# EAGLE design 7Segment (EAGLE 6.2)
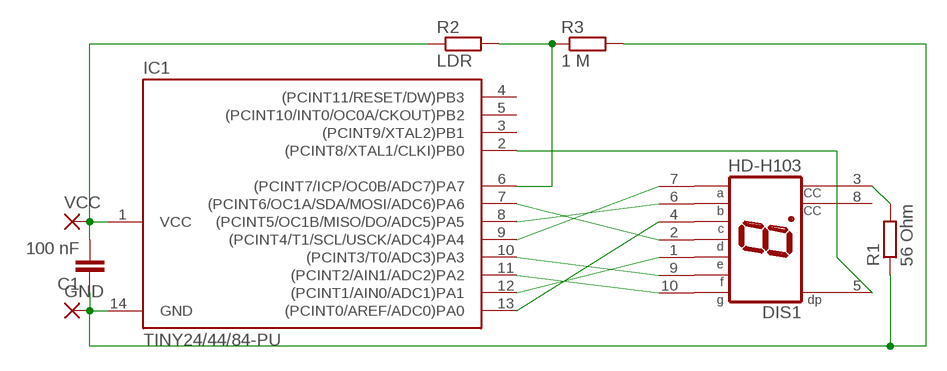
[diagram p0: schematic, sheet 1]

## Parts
C1  100 nF  C-EU025_050-025X075  [C025_050-025X075]
DIS1  HD-H103  [HDSP-M]
GND  2,15/1,0  [2,15/1,0]
IC1  TINY24/44/84-PU  [DIL14]
R1  56 Ohm  R-EU_0207/7  [0207/7]
R2  LDR  R-EU_0204/5  [0204/5]
R3  1 M  R-EU_0207/7  [0207/7]
VCC  2,15/1,0  [2,15/1,0]

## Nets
N$1: DIS1.4(C) IC1.13((PCINT0/AREF/ADC0)PA0)
N$2: C1.1 GND.1(P) IC1.14(GND) R1.1 R3.2
N$3: DIS1.1(E) IC1.12((PCINT1/AIN0/ADC1)PA1)
N$4: DIS1.10(G) IC1.11((PCINT2/AIN1/ADC2)PA2)
N$5: DIS1.9(F) IC1.10((PCINT3/T0/ADC3)PA3)
N$6: DIS1.7(A) IC1.9((PCINT4/T1/SCL/USCK/ADC4)PA4)
N$7: DIS1.6(B) IC1.8((PCINT5/OC1B/MISO/DO/ADC5)PA5)
N$8: DIS1.2(D) IC1.7((PCINT6/OC1A/SDA/MOSI/ADC6)PA6)
N$9: DIS1.5(DP) IC1.2((PCINT8/XTAL1/CLKI)PB0)
N$10: DIS1.3(CC) R1.2
N$12: IC1.6((PCINT7/ICP/OC0B/ADC7)PA7) R2.2 R3.1
VCC: C1.2 IC1.1(VCC) R2.1 VCC.1(P)
Unconnected: DIS1.8(CC) IC1.3((PCINT9/XTAL2)PB1) IC1.4((PCINT11/RESET/DW)PB3) IC1.5((PCINT10/INT0/OC0A/CKOUT)PB2)

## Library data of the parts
C1 = resistor:C-EU: CAPACITOR, European symbol
DIS1 = display-hp:HD-H103: LED DISPLAY 1-character 7 segment, decimal point right
GND VCC = wirepad:2,15/1,0: THROUGH-HOLE PAD
IC1 = avr-5:TINY24/44/84
R1-R3 = resistor:R-EU_: RESISTOR, European symbol

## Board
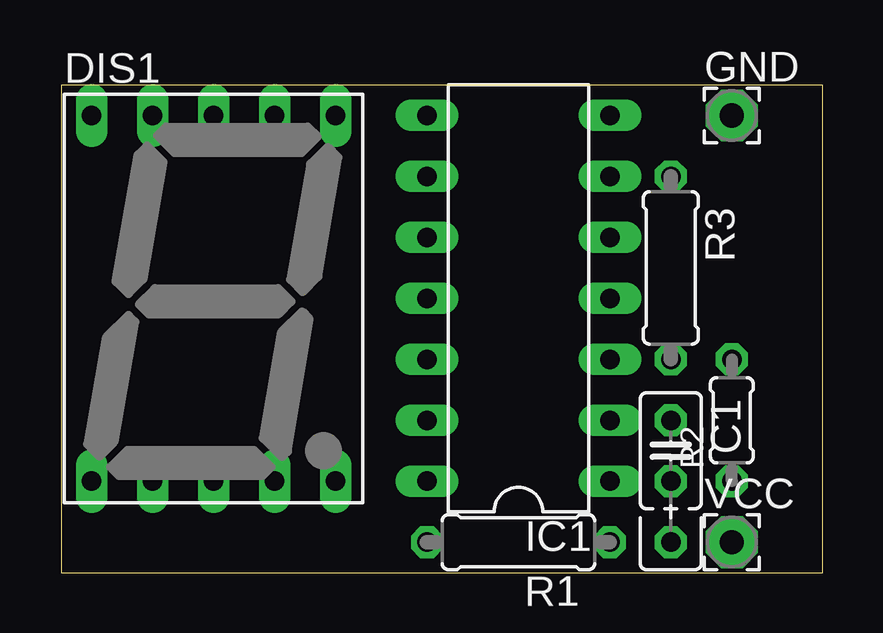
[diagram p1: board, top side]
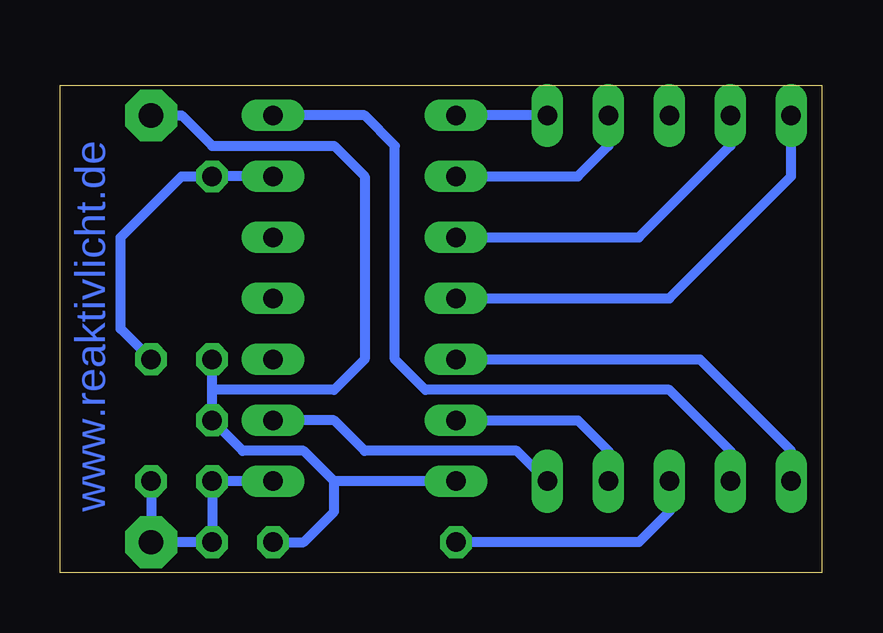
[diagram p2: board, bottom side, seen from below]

Size 31.74 x 20.31 mm. Coordinates in mm from the lower left corner, seen from the top.
Outline: 0,0 31.74,0 31.74,20.31 0,20.31 0,0
Copper layers (1*16): Top 0.035mm / dielectric 1.5mm / Bottom 0.035mm
Design rules: minimum track width 10mil, minimum drill 24mil, track to track 10mil, track to pad 10mil, pad to pad 10mil, via to via 10mil, smd to smd 10mil, copper to edge 40mil, drill to drill 8mil, minimum pad ring 10mil, minimum via ring 8mil, stop-mask expansion 4mil, vias tented up to drill 0mil, thermal gap 10mil

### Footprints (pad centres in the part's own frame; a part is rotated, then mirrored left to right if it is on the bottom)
C025_050-025X075 = drill 0.813 octagon: 1 -1.27,0; 2 1.27,0; 3 3.81,0
HDSP-M = drill 0.813 long: 1 -5.08,-7.62; 2 -2.54,-7.62; 3 0,-7.62; 4 2.54,-7.62; 5 5.08,-7.62; 6 5.08,7.62; 7 2.54,7.62; 8 0,7.62; 9 -2.54,7.62; 10 -5.08,7.62
2,15/1,0 = drill 1.016 pad 2.159 octagon: 1 0,0
DIL14 = drill 0.813 long: 1 -7.62,-3.81; 2 -5.08,-3.81; 3 -2.54,-3.81; 4 0,-3.81; 5 2.54,-3.81; 6 5.08,-3.81; 7 7.62,-3.81; 8 7.62,3.81; 9 5.08,3.81; 10 2.54,3.81; 11 0,3.81; 12 -2.54,3.81; 13 -5.08,3.81; 14 -7.62,3.81
0207/7 = drill 0.813 octagon: 1 -3.81,0; 2 3.81,0
0204/5 = drill 0.813 octagon: 1 -2.54,0; 2 2.54,0

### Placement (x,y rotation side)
C1  25.4,5.08 270 top
DIS1  6.35,11.43 0 top
GND  27.94,19.05 0 top
IC1  19.05,11.43 90 top
R1  19.05,1.27 180 top
R2  27.94,6.35 90 top
R3  25.4,12.7 270 top
VCC  27.94,1.27 0 top

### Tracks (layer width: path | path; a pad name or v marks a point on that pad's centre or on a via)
N$1
  Bottom 0.406: IC1.13 10.16,6.35 8.89,5.08 DIS1.4
N$2
  Bottom 0.406: R1.1 21.59,1.27 20.32,2.54 20.32,3.81 | IC1.14 20.32,3.81 | 20.32,3.81 21.59,5.08 24.13,5.08 C1.1 25.4,7.62 | 25.4,7.62 R3.2 | GND.1 26.67,19.05 25.4,17.78 20.32,17.78 19.05,16.51 19.05,8.89 20.32,7.62 25.4,7.62
N$3
  Bottom 0.406: IC1.12 5.08,8.89 1.27,5.08 DIS1.1
N$4
  Bottom 0.406: IC1.11 6.35,11.43 1.27,16.51 DIS1.10
N$5
  Bottom 0.406: IC1.10 7.62,13.97 3.81,17.78 DIS1.9
N$6
  Bottom 0.406: IC1.9 10.16,16.51 8.89,17.78 DIS1.7
N$7
  Bottom 0.406: DIS1.6 IC1.8
N$8
  Bottom 0.406: DIS1.2 3.81,5.08 6.35,7.62 16.51,7.62 17.78,8.89 17.78,17.78 19.05,19.05 IC1.7
N$9
  Bottom 0.406: DIS1.5 12.7,5.08 19.05,5.08 20.32,6.35 IC1.2
N$10
  Bottom 0.406: DIS1.3 6.35,2.54 7.62,1.27 R1.2
N$12
  Bottom 0.406: IC1.6 R3.1 26.67,16.51 29.21,13.97 29.21,10.16 R2.2
VCC
  Bottom 0.406: R2.1 VCC.1 25.4,1.27 C1.2 IC1.1

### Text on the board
Bottom: www.reaktivlicht.de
